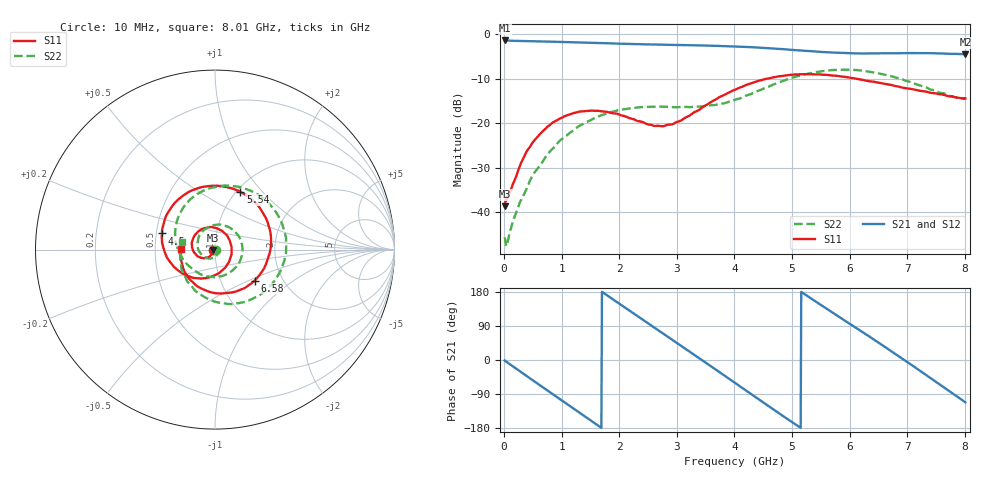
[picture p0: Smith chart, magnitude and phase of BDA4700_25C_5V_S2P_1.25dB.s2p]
!Agilent Technologies,E5071B,MY42404982,A.09.10
!Date: Mon Oct 20 13:26:33 2025
!Data & Calibration Information:
!Freq	S11:SOLT2(ON)	S21:SOLT2(ON)	S12:SOLT2(ON)	S22:SOLT2(ON)
# Hz S RI R 50
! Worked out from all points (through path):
!   801 points, 10 MHz to 8.01 GHz, reference 50 ohm
!   highest |S21| = -1.37 dB at 20 MHz (marker M1); lowest = -4.5 dB at 8.01 GHz (marker M2)
!   group delay of S21, straight-line fit = 287 ps
!   lowest |S11| = -38.7 dB at 10 MHz (marker M3), VSWR 1.02, Z = 48.9 - j0.209 ohm
!   |S11| at or under -10 dB: start of sweep to 4.56 GHz; 6.118 GHz to end of sweep
!   |S22| runs from -47.7 to -7.9 dB; largest |S21 - S12| = 0.0065
!   S11 on the Smith chart (normalised r, x): 10 MHz: 0.98, -0.00; 4.5 GHz: 0.54, +0.11; 5.54 GHz: 1.04, +0.77; 6.58 GHz: 1.44, -0.54; 8.01 GHz: 0.68, +0.00
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1e7  -0.0114 -0.00214  0.8536 -0.0185  0.8538 -0.0191  0.00509 -0.000985
2e7  -0.0125 -0.00364  0.8532 -0.0333  0.8532 -0.0362  0.00488 0.000255
3.8e8  -0.0283 -0.0368  0.6349 -0.5494  0.6346 -0.55  0.0149 -0.00947
7.2e8  -0.0735 -0.0465  0.1875 -0.8085  0.1875 -0.8088  -0.000157 -0.0415
1.03e9  -0.1167 -0.0147  -0.2756 -0.773  -0.2762 -0.773  -0.051 -0.045
1.35e9  -0.1268 0.0478  -0.6497 -0.4834  -0.6503 -0.4836  -0.0958 0.0107
1.92e9  -0.0329 0.1245  -0.7265 0.309  -0.7267 0.3093  -0.00742 0.1363
2.32e9  0.0534 0.0913  -0.3339 0.6998  -0.3339 0.7007  0.1173 0.094
2.68e9  0.092 0.0154  0.1557 0.7516  0.1557 0.7509  0.1511 -0.0271
3.36e9  0.0082 -0.1378  0.7447 0.1008  0.7459 0.1005  -0.0143 -0.1526
3.67e9  -0.0911 -0.1601  0.6751 -0.3099  0.675 -0.3118  -0.1004 -0.1253
4.01e9  -0.2103 -0.1122  0.3616 -0.6362  0.3621 -0.6361  -0.1719 -0.0628
4.5e9  -0.296 0.0899  -0.2635 -0.6538  -0.2633 -0.6552  -0.2215 0.1017
4.93e9  -0.1929 0.2884  -0.6195 -0.2659  -0.6198 -0.2688  -0.1325 0.2843
5.35e9  0.0337 0.3535  -0.6077 0.2155  -0.6084 0.2139  0.1018 0.3533
5.54e9  0.1412 0.3222  -0.4946 0.3947  -0.4952 0.3944  0.2195 0.3178
6.05e9  0.3097 0.0902  -0.0085 0.6118  -0.00873 0.6138  0.396 0.0432
6.58e9  0.2203 -0.1732  0.4835 0.3758  0.4843 0.3746  0.2538 -0.2499
6.68e9  0.1794 -0.2056  0.5419 0.2843  0.5434 0.2838  0.2011 -0.2772
7.23e9  -0.0651 -0.2217  0.5373 -0.3012  0.5375 -0.3023  -0.0762 -0.2533
7.63e9  -0.1729 -0.1171  0.1924 -0.5762  0.192 -0.5778  -0.1857 -0.1118
8.01e9  -0.19 0.00129  -0.2215 -0.5548  -0.2212 -0.5555  -0.1833 0.0438
